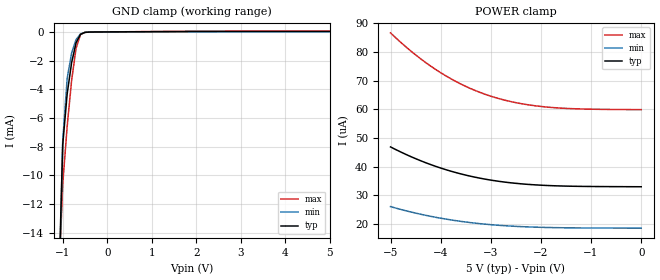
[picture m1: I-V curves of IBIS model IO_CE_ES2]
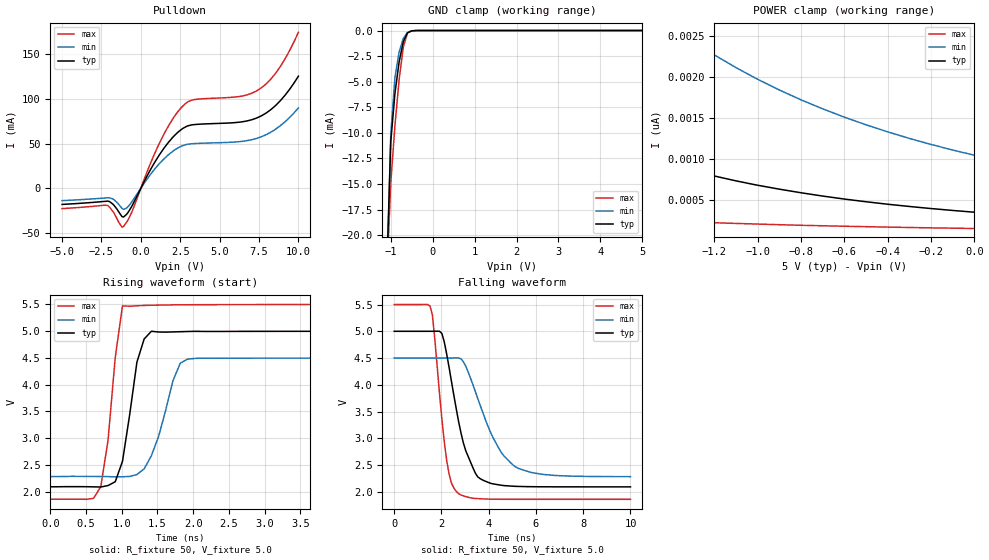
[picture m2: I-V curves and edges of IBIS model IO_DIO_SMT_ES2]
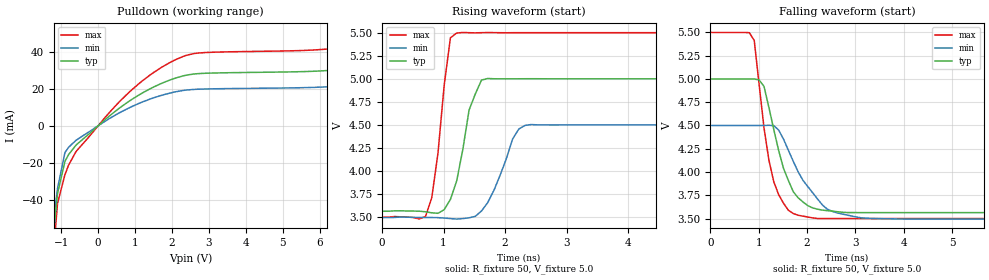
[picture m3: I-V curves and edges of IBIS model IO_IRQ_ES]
[IBIS Ver]   3.2
[Comment Char]   |_char
[File name]   r8900ce_5.ibs
[File Rev]   1.0
[Date]   2014/06/06
[Source]   This file orginated at SEIKO EPSON Corp.
[Notes]
[Disclaimer]
This information is for modeling purposes only, and is not guaranteed.
Property of SEIKO EPSON Corp.,
unauthorized reproduction and/or distribution is strictly prohibited.
[Copyright]
Copyright 2014, SEIKO EPSON Corp.
[Component]   r8900ce_5
Si_location Pin
Timing_location Pin
[Manufacturer]   SEIKO EPSON Corp.
[Package]
R_pkg   267m   NA   NA
L_pkg   2.8nH   NA   NA
C_pkg   0.70pF   NA   NA
[Pin] signal_name   model_name
1   FOE   IO_INSPD3_ES2
2   VDD   POWER
|3   VBAT   POWER2
4   FOUT   IO_OUT_ES
5   SCL   IO_INSPD2_ES2
6   CE   IO_CE_ES2
7   SDA   IO_DIO_SMT_ES2
|8   T2   TEST2
9   VSS   POWER
10   _INT   IO_IRQ_ES
| Models and submodels in the file (6): IO_CE_ES2 (Input), IO_DIO_SMT_ES2 (I/O_open_drain), IO_IRQ_ES (Open_drain), IO_INSPD3_ES2 (Input), IO_OUT_ES (3-state), IO_INSPD2_ES2 (Input)
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[Model]   IO_CE_ES2
Model_type Input
Enable Active-Low
Polarity Non-Inverting
Vinh=4.0
Vinl=1.0
C_comp   2.5p   2p   3p
[Temperature Range] 25   85   -40
[Voltage Range]   5.0   4.5   5.5
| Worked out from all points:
|   GND clamp passes 1 mA (typ) near -0.72 V on its own axis
[GND Clamp]
-5V       -765.7mA   -644.4mA   -960mA
-1.1V     -19.2mA    -20.81mA   -18.42mA
-1V       -7.873mA   -7.628mA   -10.63mA
-900mV    -4.326mA   -3.252mA   -6.591mA
-800mV    -2.147mA   -1.47mA    -3.381mA
-700mV    -761uA     -532.3uA   -1.14mA
-600mV    -166.6uA   -138.2uA   -187.5uA
-500mV    -32.82uA   -31.87uA   -30.56uA
-400mV    -10.79uA   -9.368uA   -13.23uA
5V        33.03uA    18.61uA    59.87uA
[POWER Clamp]
-5V       46.93uA    26.1uA     86.72uA
-4.7V     44.38uA    24.69uA    81.95uA
-4.5V     42.84uA    23.84uA    79.05uA
-4.3V     41.43uA    23.07uA    76.39uA
-4V       39.57uA    22.06uA    72.83uA
-3.5V     37.1uA     20.73uA    68.06uA
-3.2V     35.97uA    20.13uA    65.85uA
-2.9V     35.08uA    19.66uA    64.1uA
-2.4V     34.06uA    19.13uA    62.05uA
-1.8V     33.42uA    18.79uA    60.72uA
-1.1V     33.14uA    18.65uA    60.13uA
0V        33.03uA    18.58uA    59.93uA
[Model]   IO_DIO_SMT_ES2
Model_type I/O_open_drain
Enable Active-High
Polarity Non-Inverting
Vinh=4.0
Vinl=1.0
Vref=5.5
Vmeas=2.5
Rref=5000
C_comp   2.5p   2p   3p
[Temperature Range] 25   85   -40
[Voltage Range]   5.0   4.5   5.5
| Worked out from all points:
|   slope of the pulldown table from 0 to 0.75 V, typ, clamps not added: 29.9 ohm
|   GND clamp passes 1 mA (typ) near -0.69 V on its own axis
|   falling waveform, R_fixture 50, V_fixture 5.0: 20-80 % time 833ps typ, 1.26ns min, 486ps max; typ from 5 V to 2.09 V
|   rising waveform, R_fixture 50, V_fixture 5.0: 20-80 % time 189ps typ, 284ps min, 172ps max; typ from 2.09 V to 5 V
[Pulldown]
-5V       -18.08mA   -13.87mA   -22.75mA
-2.1V     -14.42mA   -10.67mA   -19.29mA
-1.2V     -31.63mA   -22.47mA   -43.48mA
-1.1V     -32.18mA   -23.61mA   -42.68mA
-600mV    -20.95mA   -15.86mA   -27.7mA
1.2V      37.94mA    27.96mA    51.12mA
2.6V      66.04mA    47.21mA    90.76mA
3.3V      70.95mA    49.79mA    98.77mA
6.2V      73.74mA    51.97mA    102.4mA
7.4V      78.86mA    56mA       109.3mA
8.6V      93.29mA    66.59mA    129.7mA
10V       125.2mA    89.72mA    174.2mA
[GND Clamp]
-5V       -1.008A    -841.6mA   -1.262A
-1.1V     -24.22mA   -25.63mA   -24.62mA
-1V       -10.9mA    -10.16mA   -14.91mA
-900mV    -6.131mA   -4.571mA   -9.309mA
-800mV    -3.058mA   -2.097mA   -4.786mA
-700mV    -1.078mA   -757.4uA   -1.604mA
-600mV    -224.6uA   -189.6uA   -244.1uA
-500mV    -33.81uA   -37.1uA    -22.82uA
-400mV    -4.624uA   -6.222uA   -2.07uA
5V        346.2pA    1.412nA    129.2pA
[POWER Clamp]
-5V       26.39nA    54.93nA    4.678nA
-4.4V     15.08nA    32.81nA    2.566nA
-4V       10.31nA    23.15nA    1.729nA
-3.6V     7.024nA    16.3nA     1.176nA
-3.1V     4.341nA    10.53nA    746pA
-2.6V     2.694nA    6.844nA    495.1pA
-2.5V     2.452nA    6.288nA    458.8pA
-2.3V     2.035nA    5.32nA     398.2pA
-2V       1.548nA    4.164nA    326.8pA
-1.4V     924.5pA    2.62nA     237.5pA
-700mV    543.2pA    1.607nA    180.9pA
0V        346.2pA    1.041nA    147.5pA
[Falling Waveform]
R_fixture=50
V_fixture=5.0
V_fixture_min=4.5
V_fixture_max=5.5
0s        5V         4.5V       5.5V
1.515ns   5V         4.5V       5.474V
1.616ns   5V         4.5V       5.308V
2.02ns    4.958V     4.5V       3.352V
2.222ns   4.575V     4.5V       2.586V
2.727ns   3.311V     4.501V     1.965V
3.535ns   2.281V     3.746V     1.874V
4.242ns   2.145V     2.964V     1.862V
5.051ns   2.105V     2.493V     1.86V
10ns      2.093V     2.284V     1.86V
[Rising Waveform]
R_fixture=50
V_fixture=5.0
V_fixture_min=4.5
V_fixture_max=5.5
0s        2.093V     2.283V     1.86V
707.1ps   2.089V     2.285V     2.095V
808.1ps   2.116V     2.283V     2.964V
909.1ps   2.187V     2.279V     4.512V
1.01ns    2.568V     2.279V     5.475V
1.212ns   4.423V     2.322V     5.476V
1.414ns   4.999V     2.673V     5.486V
1.717ns   4.988V     4.079V     5.493V
1.919ns   4.995V     4.479V     5.495V
10ns      5V         4.5V       5.5V
[Ramp]
R_load=50
dV/dt_r   1.744E+0/1.885E-10   1.330E+0/2.809E-10   2.184E+0/1.647E-10
dV/dt_f   1.744E+0/8.316E-10   1.330E+0/1.256E-9   2.184E+0/4.858E-10
|[End   IO_DIO_SMT_ES2
[Model]   IO_IRQ_ES
Model_type Open_drain
Enable Active-Low
Polarity Non-Inverting
Vref=5.5
Vmeas=2.5
Rref=5000
C_comp   2.5p   2p   3p
[Temperature Range] 25   85   -40
[Voltage Range]   5.0   4.5   5.5
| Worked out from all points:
|   slope of the pulldown table from 0 to 0.75 V, typ, clamps not added: 62.1 ohm
|   falling waveform, R_fixture 50, V_fixture 5.0: 20-80 % time 460ps typ, 681ps min, 335ps max; typ from 5 V to 3.56 V
|   rising waveform, R_fixture 50, V_fixture 5.0: 20-80 % time 253ps typ, 353ps min, 196ps max; typ from 3.56 V to 5 V
[Pulldown]
-5V       -904.6mA   -756.9mA   -1.133A
-1.4V     -96.77mA   -83.03mA   -118.7mA
-1.2V     -56.54mA   -50mA      -66.69mA
-1.1V     -36.82mA   -34mA      -42.05mA
-900mV    -19.32mA   -14.56mA   -26.52mA
-800mV    -15.63mA   -11.64mA   -21.32mA
800mV     12.78mA    9.33mA     17.43mA
2.3V      27.02mA    19.12mA    37.54mA
7.1V      31.97mA    22.61mA    44.55mA
8.2V      38.14mA    26.96mA    53.64mA
9.5V      52.39mA    36.93mA    74.29mA
10V       59.96mA    42.26mA    85.06mA
[Falling Waveform]
R_fixture=50
V_fixture=5.0
V_fixture_min=4.5
V_fixture_max=5.5
0s        5V         4.5V       5.5V
808.1ps   5V         4.5V       5.497V
909.1ps   5V         4.5V       5.414V
1.111ns   4.92V      4.5V       4.474V
1.313ns   4.457V     4.498V     3.896V
1.515ns   4.038V     4.353V     3.664V
1.717ns   3.788V     4.114V     3.554V
2.424ns   3.584V     3.599V     3.499V
3.131ns   3.564V     3.507V     3.499V
10ns      3.563V     3.494V     3.499V
[Rising Waveform]
R_fixture=50
V_fixture=5.0
V_fixture_min=4.5
V_fixture_max=5.5
0s        3.563V     3.494V     3.499V
707.1ps   3.558V     3.496V     3.508V
808.1ps   3.547V     3.496V     3.711V
909.1ps   3.541V     3.494V     4.194V
1.111ns   3.692V     3.484V     5.444V
1.212ns   3.891V     3.479V     5.496V
1.414ns   4.66V      3.493V     5.5V
1.717ns   5.003V     3.657V     5.501V
2.323ns   5V         4.495V     5.5V
10ns      5V         4.5V       5.5V
[Ramp]
R_load=50
dV/dt_r   8.619E-1/2.450E-10   6.035E-1/3.433E-10   1.201E+0/1.901E-10
dV/dt_f   8.619E-1/4.558E-10   6.035E-1/6.797E-10   1.201E+0/3.342E-10
|[End   IO_IRQ_ES
